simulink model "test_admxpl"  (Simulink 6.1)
settings: Solver=ode45  StartTime=0.0  StopTime=400  RelTol=1e-3
undefined symbols (not defined in the file or in its folder): Bit, Location, Lower, netlist, Width
libraries: xbsIndex_r3 x92, adlibrary2 x3

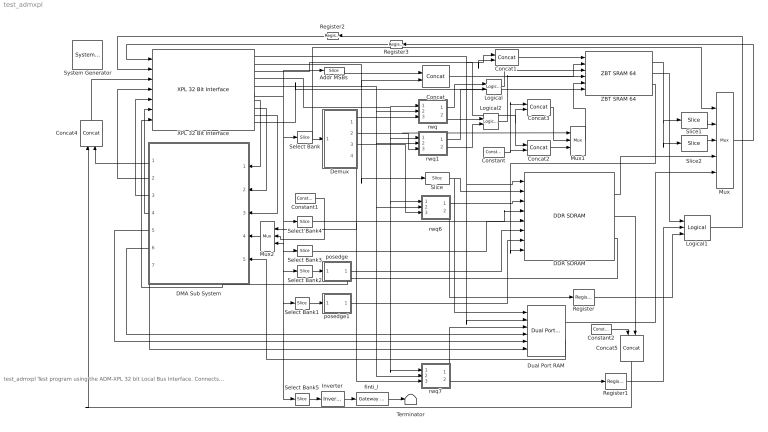
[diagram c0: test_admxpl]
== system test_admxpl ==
  note: test_admxpl Test program using the ADM-XPL 32 bit Local Bus Interface. Connects to the ZBT SRAM and DDR SDRAM
  " System Generator" : xbsIndex_r3/ System Generator  Tag=genX  xilinxfamily=Virtex2P  part=xc2vp30  speed=-5  package=ff896  synthesis_tool=XST  directory=./netlist  testbench=off  simulink_period=1  sysclk_period=10  incr_netlist=off  trim_vbits=Everywhere in SubSystem  dbl_ovrd=According to Block Masks  core_generation=According to Block Masks  run_coregen=off  deprecated_control=off  eval_field=0
  Addr MSBs : xbsIndex_r3/Slice  mode=Lower Bit Location + Width  nbits=4  bit1=0  base1=MSB of Input  bit0=4  base0=LSB of Input  boolean_output=off  explicit_period=on  period=1  dbl_ovrd=off
  Concat : xbsIndex_r3/Concat  num_inputs=2  explicit_period=on  period=1  dbl_ovrd=off
  Concat1 : xbsIndex_r3/Concat  num_inputs=2  explicit_period=on  period=1  dbl_ovrd=off
  Concat2 : xbsIndex_r3/Concat  num_inputs=2  explicit_period=off  period=1  dbl_ovrd=off
  Concat3 : xbsIndex_r3/Concat  num_inputs=2  explicit_period=off  period=1  dbl_ovrd=off
  Concat4 : xbsIndex_r3/Concat  Orientation=up  num_inputs=2  explicit_period=on  period=1  dbl_ovrd=off
  Concat5 : xbsIndex_r3/Concat  Orientation=down  num_inputs=2  explicit_period=on  period=1  dbl_ovrd=off
  Constant : xbsIndex_r3/Constant  const=0  equ=P=C  arith_type=Unsigned  n_bits=4  bin_pt=0  opselect=C  inp2=PCIN>>17  opr=+  inp1=P  carry=CIN  iostate=0  explicit_period=off  period=1  dbl_ovrd=off
  Constant1 : xbsIndex_r3/Constant  const=0  equ=P=C  arith_type=Unsigned  n_bits=32  bin_pt=0  opselect=C  inp2=PCIN>>17  opr=+  inp1=P  carry=CIN  iostate=0  explicit_period=off  period=1  dbl_ovrd=off
  Constant2 : xbsIndex_r3/Constant  const=0  equ=P=C  arith_type=Unsigned  n_bits=3  bin_pt=0  opselect=C  inp2=PCIN>>17  opr=+  inp1=P  carry=CIN  iostate=0  explicit_period=off  period=1  dbl_ovrd=off
  DDR SDRAM : adlibrary2/ADM-XPL/DDR SDRAM  memsize=1
  DMA Sub System : Subsystem  Orientation=left
  Demux : Subsystem
  Dual Port RAM : xbsIndex_r3/Dual Port RAM  depth=1024  initVector=sin(pi*(0:15)/16)  write_mode_A=Read After Write  write_mode_B=Read After Write  latency=1  mem_collision=off  init_zero=on  explicit_period=on  period=1  dbl_ovrd=off  rst_a=off  init_a=0  rst_b=off  init_b=0  show_param=off  distributed_mem=off  use_rpm=off  gen_core=off
  Inverter : xbsIndex_r3/Inverter  latency=0  explicit_period=off  period=1  en=off  dbl_ovrd=off  show_param=off
  Logical : xbsIndex_r3/Logical  logical_function=OR  inputs=2  precision=Full  arith_type=Unsigned  n_bits=8  bin_pt=2  align_bp=on  latency=0  explicit_period=off  period=1  en=off  dbl_ovrd=off  show_param=off
  Logical1 : xbsIndex_r3/Logical  logical_function=OR  inputs=3  precision=Full  arith_type=Unsigned  n_bits=8  bin_pt=2  align_bp=on  latency=0  explicit_period=off  period=1  en=off  dbl_ovrd=off  show_param=off
  Logical2 : xbsIndex_r3/Logical  logical_function=OR  inputs=2  precision=Full  arith_type=Unsigned  n_bits=8  bin_pt=2  align_bp=on  latency=0  explicit_period=off  period=1  en=off  dbl_ovrd=off  show_param=off
  Mux : xbsIndex_r3/Mux  inputs=4  precision=Full  arith_type="Signed  (2's comp)"  n_bits=8  bin_pt=2  quantization=Truncate  overflow=Wrap  latency=0  explicit_period=off  period=1  en=off  dbl_ovrd=off  show_param=off  mux_type=off  use_rpm=off  gen_core=off
  Mux1 : xbsIndex_r3/Mux  inputs=2  precision=Full  arith_type="Signed  (2's comp)"  n_bits=8  bin_pt=2  quantization=Truncate  overflow=Wrap  latency=0  explicit_period=off  period=1  en=off  dbl_ovrd=off  show_param=off  mux_type=off  use_rpm=off  gen_core=off
  Mux2 : xbsIndex_r3/Mux  Orientation=left  inputs=2  precision=Full  arith_type="Signed  (2's comp)"  n_bits=8  bin_pt=2  quantization=Truncate  overflow=Wrap  latency=0  explicit_period=off  period=1  en=off  dbl_ovrd=off  show_param=off  mux_type=off  use_rpm=off  gen_core=off
  Register : xbsIndex_r3/Register  init=0  reg_only_valid=off  explicit_period=off  period=1  rst=off  en=off  out_en=off  dbl_ovrd=off  show_param=off
  Register1 : xbsIndex_r3/Register  init=0  reg_only_valid=off  explicit_period=off  period=1  rst=off  en=off  out_en=off  dbl_ovrd=off  show_param=off
  Register2 : xbsIndex_r3/Register  Orientation=left  init=0  reg_only_valid=off  explicit_period=on  period=1  rst=off  en=off  out_en=off  dbl_ovrd=off  show_param=off
  Register3 : xbsIndex_r3/Register  Orientation=left  init=0  reg_only_valid=off  explicit_period=on  period=1  rst=off  en=off  out_en=off  dbl_ovrd=off  show_param=off
  Select Bank : xbsIndex_r3/Slice  mode=Lower Bit Location + Width  nbits=2  bit1=0  base1=MSB of Input  bit0=0  base0=LSB of Input  boolean_output=off  explicit_period=on  period=1  dbl_ovrd=off
  Select Bank1 : xbsIndex_r3/Slice  mode=Lower Bit Location + Width  nbits=1  bit1=0  base1=MSB of Input  bit0=3  base0=LSB of Input  boolean_output=on  explicit_period=on  period=1  dbl_ovrd=off
  Select Bank2 : xbsIndex_r3/Slice  mode=Lower Bit Location + Width  nbits=1  bit1=0  base1=MSB of Input  bit0=2  base0=LSB of Input  boolean_output=on  explicit_period=on  period=1  dbl_ovrd=off
  Select Bank3 : xbsIndex_r3/Slice  mode=Lower Bit Location + Width  nbits=4  bit1=0  base1=MSB of Input  bit0=8  base0=LSB of Input  boolean_output=off  explicit_period=on  period=1  dbl_ovrd=off
  Select Bank4 : xbsIndex_r3/Slice  mode=Lower Bit Location + Width  nbits=15  bit1=0  base1=MSB of Input  bit0=16  base0=LSB of Input  boolean_output=off  explicit_period=on  period=1  dbl_ovrd=off
  Select Bank5 : xbsIndex_r3/Slice  mode=Lower Bit Location + Width  nbits=1  bit1=0  base1=MSB of Input  bit0=15  base0=LSB of Input  boolean_output=on  explicit_period=on  period=1  dbl_ovrd=off
  Slice : xbsIndex_r3/Slice  mode=Lower Bit Location + Width  nbits=10  bit1=0  base1=MSB of Input  bit0=0  base0=LSB of Input  boolean_output=off  explicit_period=on  period=1  dbl_ovrd=off
  Slice1 : xbsIndex_r3/Slice  mode=Lower Bit Location + Width  nbits=32  bit1=0  base1=MSB of Input  bit0=0  base0=LSB of Input  boolean_output=off  explicit_period=off  period=1  dbl_ovrd=off
  Slice2 : xbsIndex_r3/Slice  mode=Lower Bit Location + Width  nbits=32  bit1=0  base1=MSB of Input  bit0=32  base0=LSB of Input  boolean_output=off  explicit_period=off  period=1  dbl_ovrd=off
  Terminator : Terminator
  XPL 32 Bit Interface : adlibrary2/ADM-XPL/XPL 32 Bit Interface  program='load test_admxpl_ddr_program.txt'  clock_ratio=1.5
  ZBT SRAM 64 : adlibrary2/ADM-XPL/ZBT SRAM 64
  finti_l : xbsIndex_r3/Gateway Out  output_type=Double  nbits=8  bin_pt=6  arith_type=Boolean  quantization=Truncate  overflow=Wrap  hdl_port=on  timing_constraint=None  locs_specified=on  LOCs={'G26'}  needs_fixed_name=off  show_param=off
  posedge : Subsystem
  posedge1 : Subsystem
  rwq : Subsystem
  rwq1 : Subsystem
  rwq6 : Subsystem
  rwq7 : Subsystem
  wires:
  XPL 32 Bit Interface/1 -> Concat1/1, Concat1/2, Dual Port RAM/2, DDR SDRAM/1
  Register/1 -> Logical1/3
  Register1/1 -> Logical1/2
  Mux/1 -> Register3/1
  Register2/1 -> XPL 32 Bit Interface/2
  Register3/1 -> XPL 32 Bit Interface/1
  Slice/1 -> Dual Port RAM/1, DDR SDRAM/2
  Addr MSBs/1 -> Concat/1
  XPL 32 Bit Interface/2 -> Concat/2, Slice/1
  Select Bank/1 -> Demux/1(Select), Mux/1
  rwq6/1(wq) -> DDR SDRAM/3
  rwq6/2(rq) -> Register/1
  rwq7/1(wq) -> Dual Port RAM/3
  rwq7/2(rq) -> Register1/1
  Demux/1(En0) -> rwq/3(e)
  Demux/2(En1) -> rwq1/3(e), Mux1/1
  DMA Sub System/2(Read IFIFO) -> XPL 32 Bit Interface/4
  DMA Sub System/3(Write OFIFO) -> XPL 32 Bit Interface/5
  DMA Sub System/4(OFIFO_Data) -> XPL 32 Bit Interface/6
  Dual Port RAM/2 -> DMA Sub System/5(DP_RAM_Data)
  DMA Sub System/7(DP_RAM_WE) -> Dual Port RAM/6
  DMA Sub System/6(DP_RAM_Addr) -> Dual Port RAM/4
  DMA Sub System/5(DP_RAM_WData) -> Dual Port RAM/5
  Logical1/1 -> Register2/1
  rwq/1(wq) -> Logical/1
  rwq1/1(wq) -> Logical/2
  rwq/2(rq) -> Logical2/1
  rwq1/2(rq) -> Logical2/2
  Demux/3(En2) -> rwq6/3(e)
  Demux/4(En3) -> rwq7/3(e), Mux2/1
  DDR SDRAM/1 -> Mux/4
  Dual Port RAM/1 -> Mux/5
  XPL 32 Bit Interface/4 -> rwq/1(w), rwq1/1(w), rwq6/1(w), rwq7/1(w)
  XPL 32 Bit Interface/9 -> DMA Sub System/3(OFIFO_Full)
  XPL 32 Bit Interface/8 -> DMA Sub System/2(IFIFO_Empty)
  XPL 32 Bit Interface/7 -> DMA Sub System/1(IFIFO_Data)
  XPL 32 Bit Interface/6 -> Select Bank4/1, Select Bank2/1, Select Bank1/1, Select Bank5/1, Select Bank3/1, Mux2/3, Select Bank/1, Addr MSBs/1
  XPL 32 Bit Interface/5 -> rwq7/2(r), rwq6/2(r), rwq1/2(r), rwq/2(r)
  Concat/1 -> ZBT SRAM 64/2
  Concat1/1 -> ZBT SRAM 64/1
  Logical/1 -> ZBT SRAM 64/3
  Logical2/1 -> ZBT SRAM 64/4
  Slice1/1 -> Mux/2
  Slice2/1 -> Mux/3
  ZBT SRAM 64/1 -> Slice1/1, Slice2/1
  ZBT SRAM 64/2 -> Logical1/1
  Mux1/1 -> ZBT SRAM 64/5
  Concat3/1 -> Mux1/2
  Concat2/1 -> Mux1/3
  XPL 32 Bit Interface/3 -> Concat2/1, Concat3/2
  Constant/1 -> Concat2/2, Concat3/1
  Concat4/1 -> XPL 32 Bit Interface/3
  DMA Sub System/1(Status) -> Concat4/2
  DDR SDRAM/2 -> Concat5/2
  Concat5/1 -> Concat4/1
  posedge/1(Out1) -> DDR SDRAM/6
  posedge1/1(Out1) -> DDR SDRAM/7
  Select Bank2/1 -> posedge/1(In1)
  Select Bank1/1 -> posedge1/1(In1)
  Select Bank3/1 -> DDR SDRAM/5
  Select Bank4/1 -> DDR SDRAM/4
  Select Bank5/1 -> Inverter/1
  finti_l/1 -> Terminator/1
  Mux2/1 -> DMA Sub System/4(Control)
  Constant1/1 -> Mux2/2
  XPL 32 Bit Interface/10 -> ZBT SRAM 64/6
  Constant2/1 -> Concat5/1
  ZBT SRAM 64/3 -> DDR SDRAM/8
  DDR SDRAM/3 -> XPL 32 Bit Interface/7
  Inverter/1 -> finti_l/1

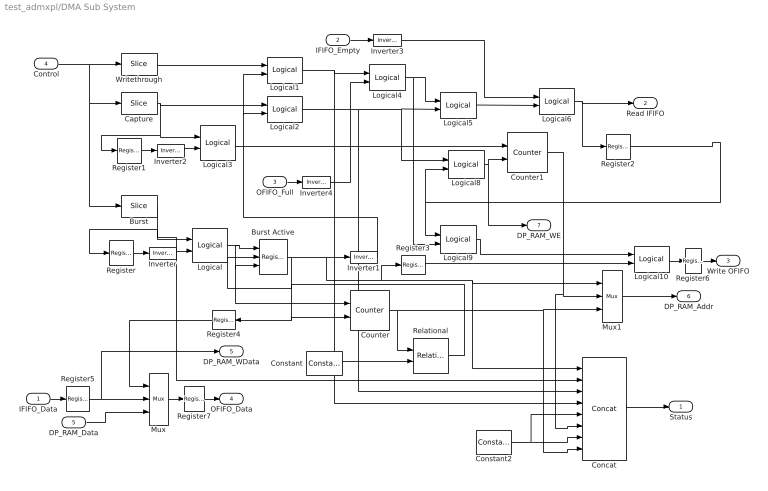
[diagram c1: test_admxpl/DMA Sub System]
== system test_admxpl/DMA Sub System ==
  IFIFO_Data : Inport  Port=1  LatchInput=off
  IFIFO_Empty : Inport  Port=2  LatchInput=off
  OFIFO_Full : Inport  Port=3  LatchInput=off
  Control : Inport  Port=4  LatchInput=off
  DP_RAM_Data : Inport  Port=5  LatchInput=off
  Burst : xbsIndex_r3/Slice  mode=Lower Bit Location + Width  nbits=1  bit1=0  base1=MSB of Input  bit0=6  base0=LSB of Input  boolean_output=on  explicit_period=on  period=1  dbl_ovrd=off
  Burst Active : xbsIndex_r3/Register  init=0  reg_only_valid=off  explicit_period=on  period=1  rst=on  en=on  out_en=off  dbl_ovrd=off  show_param=off
  Capture : xbsIndex_r3/Slice  mode=Lower Bit Location + Width  nbits=1  bit1=0  base1=MSB of Input  bit0=5  base0=LSB of Input  boolean_output=on  explicit_period=on  period=1  dbl_ovrd=off
  Concat : xbsIndex_r3/Concat  num_inputs=8  explicit_period=on  period=1  dbl_ovrd=off
  Constant : xbsIndex_r3/Constant  const=511  equ=P=C  arith_type=Unsigned  n_bits=10  bin_pt=0  opselect=C  inp2=PCIN>>17  opr=+  inp1=P  carry=CIN  iostate=0  explicit_period=off  period=1  dbl_ovrd=off
  Constant2 : xbsIndex_r3/Constant  const=0  equ=P=C  arith_type=Unsigned  n_bits=2  bin_pt=0  opselect=C  inp2=PCIN>>17  opr=+  inp1=P  carry=CIN  iostate=0  explicit_period=off  period=1  dbl_ovrd=off
  Counter : xbsIndex_r3/Counter  cnt_type=Count Limited  n_bits=10  bin_pt=0  arith_type=Unsigned  start_count=0  cnt_to=Inf  cnt_by_val=1  operation=Up  explicit_period=on  period=1  load_pin=off  rst=on  en=on  dbl_ovrd=off  show_param=off  use_rpm=on  gen_core=off
  Counter1 : xbsIndex_r3/Counter  cnt_type=Count Limited  n_bits=10  bin_pt=0  arith_type=Unsigned  start_count=0  cnt_to=Inf  cnt_by_val=1  operation=Up  explicit_period=on  period=1  load_pin=off  rst=on  en=on  dbl_ovrd=off  show_param=off  use_rpm=on  gen_core=off
  Inverter{,1..2,4} (4 alike) : xbsIndex_r3/Inverter  latency=0  explicit_period=off  period=1  en=off  dbl_ovrd=off  show_param=off
  Inverter3 : xbsIndex_r3/Inverter  latency=0  explicit_period=on  period=1  en=off  dbl_ovrd=off  show_param=off
  Logical : xbsIndex_r3/Logical  logical_function=AND  inputs=2  precision=Full  arith_type=Unsigned  n_bits=8  bin_pt=2  align_bp=on  latency=0  explicit_period=on  period=1  en=off  dbl_ovrd=off  show_param=off
  Logical{1..2,4,8..9} (5 alike) : xbsIndex_r3/Logical  logical_function=AND  inputs=2  precision=Full  arith_type=Unsigned  n_bits=8  bin_pt=2  align_bp=on  latency=0  explicit_period=off  period=1  en=off  dbl_ovrd=off  show_param=off
  Logical10 : xbsIndex_r3/Logical  logical_function=OR  inputs=2  precision=Full  arith_type=Unsigned  n_bits=8  bin_pt=2  align_bp=on  latency=0  explicit_period=on  period=1  en=off  dbl_ovrd=off  show_param=off
  Logical3 : xbsIndex_r3/Logical  logical_function=AND  inputs=2  precision=Full  arith_type=Unsigned  n_bits=8  bin_pt=2  align_bp=on  latency=0  explicit_period=on  period=1  en=off  dbl_ovrd=off  show_param=off
  Logical5 : xbsIndex_r3/Logical  logical_function=OR  inputs=2  precision=Full  arith_type=Unsigned  n_bits=8  bin_pt=2  align_bp=on  latency=0  explicit_period=off  period=1  en=off  dbl_ovrd=off  show_param=off
  Logical6 : xbsIndex_r3/Logical  logical_function=AND  inputs=2  precision=Full  arith_type=Unsigned  n_bits=8  bin_pt=2  align_bp=on  latency=0  explicit_period=on  period=1  en=off  dbl_ovrd=off  show_param=off
  Mux : xbsIndex_r3/Mux  inputs=2  precision=Full  arith_type="Signed  (2's comp)"  n_bits=8  bin_pt=2  quantization=Truncate  overflow=Wrap  latency=0  explicit_period=on  period=1  en=off  dbl_ovrd=off  show_param=off  mux_type=off  use_rpm=off  gen_core=off
  Mux1 : xbsIndex_r3/Mux  inputs=2  precision=Full  arith_type="Signed  (2's comp)"  n_bits=8  bin_pt=2  quantization=Truncate  overflow=Wrap  latency=0  explicit_period=off  period=1  en=off  dbl_ovrd=off  show_param=off  mux_type=off  use_rpm=off  gen_core=off
  Register{,1..3,5..7} (7 alike) : xbsIndex_r3/Register  init=0  reg_only_valid=off  explicit_period=on  period=1  rst=off  en=off  out_en=off  dbl_ovrd=off  show_param=off
  Register4 : xbsIndex_r3/Register  Orientation=left  init=0  reg_only_valid=off  explicit_period=on  period=1  rst=off  en=off  out_en=off  dbl_ovrd=off  show_param=off
  Relational : xbsIndex_r3/Relational  mode=a=b  latency=0  explicit_period=off  period=1  en=off  dbl_ovrd=off  show_param=off
  Writethrough : xbsIndex_r3/Slice  mode=Lower Bit Location + Width  nbits=1  bit1=0  base1=MSB of Input  bit0=4  base0=LSB of Input  boolean_output=on  explicit_period=on  period=1  dbl_ovrd=off
  Status : Outport
  Read IFIFO : Outport  Port=2
  Write OFIFO : Outport  Port=3
  OFIFO_Data : Outport  Port=4
  DP_RAM_WData : Outport  Port=5
  DP_RAM_Addr : Outport  Port=6
  DP_RAM_WE : Outport  Port=7
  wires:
  Mux/1 -> Register7/1
  IFIFO_Data/1 -> Register5/1
  DP_RAM_Data/1 -> Mux/3
  Control/1 -> Writethrough/1, Burst/1, Capture/1
  Burst/1 -> Register/1, Logical/1, Concat/2
  Register/1 -> Inverter/1
  Inverter/1 -> Logical/2
  Logical/1 -> Burst Active/1, Burst Active/3, Counter/1
  Burst Active/1 -> Inverter1/1, Register3/1, Mux1/1, Concat/1, Counter/2, Register4/1
  Inverter1/1 -> Logical1/2, Logical2/2
  Capture/1 -> Logical2/1, Logical3/1, Register1/1
  Writethrough/1 -> Logical1/1
  Register1/1 -> Inverter2/1
  Inverter2/1 -> Logical3/2
  Logical3/1 -> Counter1/1
  IFIFO_Empty/1 -> Inverter3/1
  OFIFO_Full/1 -> Inverter4/1
  Logical1/1 -> Logical4/1, Concat/4
  Inverter4/1 -> Logical4/2
  Logical2/1 -> Logical5/2, Logical8/1, Concat/3
  Logical4/1 -> Logical5/1, Logical9/2
  Inverter3/1 -> Logical6/1
  Logical5/1 -> Logical6/2
  Logical6/1 -> Read IFIFO/1, Register2/1
  Register2/1 -> Logical8/2, Logical9/1
  Logical8/1 -> Counter1/2, DP_RAM_WE/1
  Mux1/1 -> DP_RAM_Addr/1
  Counter1/1 -> Mux1/2, Concat/6
  Counter/1 -> Relational/1, Mux1/3, Concat/8
  Logical9/1 -> Logical10/1
  Register3/1 -> Logical10/2
  Constant/1 -> Relational/2
  Relational/1 -> Burst Active/2
  Constant2/1 -> Concat/5, Concat/7
  Concat/1 -> Status/1
  Logical10/1 -> Register6/1
  Register4/1 -> Mux/1
  Register5/1 -> Mux/2, DP_RAM_WData/1
  Register6/1 -> Write OFIFO/1
  Register7/1 -> OFIFO_Data/1

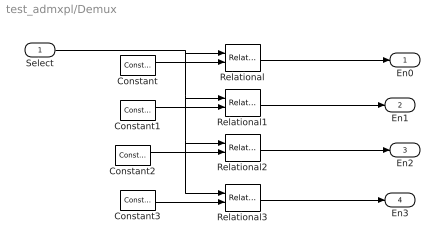
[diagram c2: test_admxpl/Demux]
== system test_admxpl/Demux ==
  Select : Inport  Port=1  LatchInput=off
  Constant : xbsIndex_r3/Constant  const=0  equ=P=C  arith_type=Unsigned  n_bits=2  bin_pt=0  opselect=C  inp2=PCIN>>17  opr=+  inp1=P  carry=CIN  iostate=0  explicit_period=off  period=1  dbl_ovrd=off
  Constant1 : xbsIndex_r3/Constant  const=1  equ=P=C  arith_type=Unsigned  n_bits=2  bin_pt=0  opselect=C  inp2=PCIN>>17  opr=+  inp1=P  carry=CIN  iostate=0  explicit_period=off  period=1  dbl_ovrd=off
  Constant2 : xbsIndex_r3/Constant  const=2  equ=P=C  arith_type=Unsigned  n_bits=2  bin_pt=0  opselect=C  inp2=PCIN>>17  opr=+  inp1=P  carry=CIN  iostate=0  explicit_period=off  period=1  dbl_ovrd=off
  Constant3 : xbsIndex_r3/Constant  const=3  equ=P=C  arith_type=Unsigned  n_bits=2  bin_pt=0  opselect=C  inp2=PCIN>>17  opr=+  inp1=P  carry=CIN  iostate=0  explicit_period=off  period=1  dbl_ovrd=off
  Relational{,1..3} (4 alike) : xbsIndex_r3/Relational  mode=a=b  latency=0  explicit_period=off  period=1  en=off  dbl_ovrd=off  show_param=off
  En0 : Outport
  En1 : Outport  Port=2
  En2 : Outport  Port=3
  En3 : Outport  Port=4
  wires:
  Relational/1 -> En0/1
  Relational1/1 -> En1/1
  Relational2/1 -> En2/1
  Relational3/1 -> En3/1
  Select/1 -> Relational/1, Relational1/1, Relational2/1, Relational3/1
  Constant/1 -> Relational/2
  Constant1/1 -> Relational1/2
  Constant2/1 -> Relational2/2
  Constant3/1 -> Relational3/2

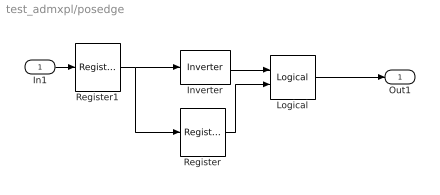
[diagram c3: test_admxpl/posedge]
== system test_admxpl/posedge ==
  In1 : Inport  Port=1  LatchInput=off
  Inverter : xbsIndex_r3/Inverter  latency=0  explicit_period=off  period=1  en=off  dbl_ovrd=off  show_param=off
  Logical : xbsIndex_r3/Logical  logical_function=AND  inputs=2  precision=Full  arith_type=Unsigned  n_bits=8  bin_pt=2  align_bp=on  latency=0  explicit_period=off  period=1  en=off  dbl_ovrd=off  show_param=off
  Register : xbsIndex_r3/Register  init=0  reg_only_valid=off  explicit_period=on  period=1  rst=off  en=off  out_en=off  dbl_ovrd=off  show_param=off
  Register1 : xbsIndex_r3/Register  init=0  reg_only_valid=off  explicit_period=on  period=1  rst=off  en=off  out_en=off  dbl_ovrd=off  show_param=off
  Out1 : Outport
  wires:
  Inverter/1 -> Logical/1
  Logical/1 -> Out1/1
  Register/1 -> Logical/2
  In1/1 -> Register1/1
  Register1/1 -> Inverter/1, Register/1

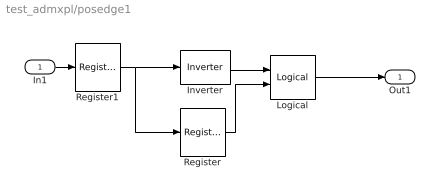
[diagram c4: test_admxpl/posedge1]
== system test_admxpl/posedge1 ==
  In1 : Inport  Port=1  LatchInput=off
  Inverter : xbsIndex_r3/Inverter  latency=0  explicit_period=off  period=1  en=off  dbl_ovrd=off  show_param=off
  Logical : xbsIndex_r3/Logical  logical_function=AND  inputs=2  precision=Full  arith_type=Unsigned  n_bits=8  bin_pt=2  align_bp=on  latency=0  explicit_period=off  period=1  en=off  dbl_ovrd=off  show_param=off
  Register : xbsIndex_r3/Register  init=0  reg_only_valid=off  explicit_period=on  period=1  rst=off  en=off  out_en=off  dbl_ovrd=off  show_param=off
  Register1 : xbsIndex_r3/Register  init=0  reg_only_valid=off  explicit_period=on  period=1  rst=off  en=off  out_en=off  dbl_ovrd=off  show_param=off
  Out1 : Outport
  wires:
  Inverter/1 -> Logical/1
  Logical/1 -> Out1/1
  Register/1 -> Logical/2
  In1/1 -> Register1/1
  Register1/1 -> Inverter/1, Register/1

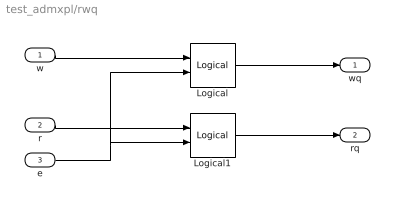
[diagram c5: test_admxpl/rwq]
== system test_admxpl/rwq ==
  w : Inport  Port=1  LatchInput=off
  r : Inport  Port=2  LatchInput=off
  e : Inport  Port=3  LatchInput=off
  Logical : xbsIndex_r3/Logical  logical_function=AND  inputs=2  precision=Full  arith_type=Unsigned  n_bits=8  bin_pt=2  align_bp=on  latency=0  explicit_period=off  period=1  en=off  dbl_ovrd=off  show_param=off
  Logical1 : xbsIndex_r3/Logical  logical_function=AND  inputs=2  precision=Full  arith_type=Unsigned  n_bits=8  bin_pt=2  align_bp=on  latency=0  explicit_period=off  period=1  en=off  dbl_ovrd=off  show_param=off
  wq : Outport
  rq : Outport  Port=2
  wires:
  e/1 -> Logical1/2, Logical/2
  r/1 -> Logical1/1
  w/1 -> Logical/1
  Logical/1 -> wq/1
  Logical1/1 -> rq/1

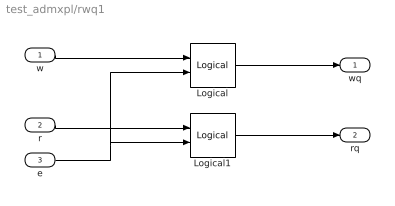
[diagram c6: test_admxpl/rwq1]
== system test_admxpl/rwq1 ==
  w : Inport  Port=1  LatchInput=off
  r : Inport  Port=2  LatchInput=off
  e : Inport  Port=3  LatchInput=off
  Logical : xbsIndex_r3/Logical  logical_function=AND  inputs=2  precision=Full  arith_type=Unsigned  n_bits=8  bin_pt=2  align_bp=on  latency=0  explicit_period=off  period=1  en=off  dbl_ovrd=off  show_param=off
  Logical1 : xbsIndex_r3/Logical  logical_function=AND  inputs=2  precision=Full  arith_type=Unsigned  n_bits=8  bin_pt=2  align_bp=on  latency=0  explicit_period=off  period=1  en=off  dbl_ovrd=off  show_param=off
  wq : Outport
  rq : Outport  Port=2
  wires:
  e/1 -> Logical1/2, Logical/2
  r/1 -> Logical1/1
  w/1 -> Logical/1
  Logical/1 -> wq/1
  Logical1/1 -> rq/1

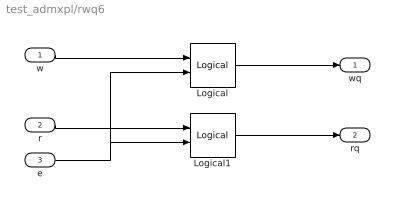
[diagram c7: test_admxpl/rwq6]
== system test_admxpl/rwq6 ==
  w : Inport  Port=1  LatchInput=off
  r : Inport  Port=2  LatchInput=off
  e : Inport  Port=3  LatchInput=off
  Logical : xbsIndex_r3/Logical  logical_function=AND  inputs=2  precision=Full  arith_type=Unsigned  n_bits=8  bin_pt=2  align_bp=on  latency=0  explicit_period=off  period=1  en=off  dbl_ovrd=off  show_param=off
  Logical1 : xbsIndex_r3/Logical  logical_function=AND  inputs=2  precision=Full  arith_type=Unsigned  n_bits=8  bin_pt=2  align_bp=on  latency=0  explicit_period=off  period=1  en=off  dbl_ovrd=off  show_param=off
  wq : Outport
  rq : Outport  Port=2
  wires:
  e/1 -> Logical1/2, Logical/2
  r/1 -> Logical1/1
  w/1 -> Logical/1
  Logical/1 -> wq/1
  Logical1/1 -> rq/1

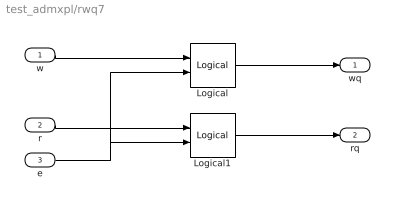
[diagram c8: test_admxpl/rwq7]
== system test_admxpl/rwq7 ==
  w : Inport  Port=1  LatchInput=off
  r : Inport  Port=2  LatchInput=off
  e : Inport  Port=3  LatchInput=off
  Logical : xbsIndex_r3/Logical  logical_function=AND  inputs=2  precision=Full  arith_type=Unsigned  n_bits=8  bin_pt=2  align_bp=on  latency=0  explicit_period=off  period=1  en=off  dbl_ovrd=off  show_param=off
  Logical1 : xbsIndex_r3/Logical  logical_function=AND  inputs=2  precision=Full  arith_type=Unsigned  n_bits=8  bin_pt=2  align_bp=on  latency=0  explicit_period=off  period=1  en=off  dbl_ovrd=off  show_param=off
  wq : Outport
  rq : Outport  Port=2
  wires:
  e/1 -> Logical1/2, Logical/2
  r/1 -> Logical1/1
  w/1 -> Logical/1
  Logical/1 -> wq/1
  Logical1/1 -> rq/1
